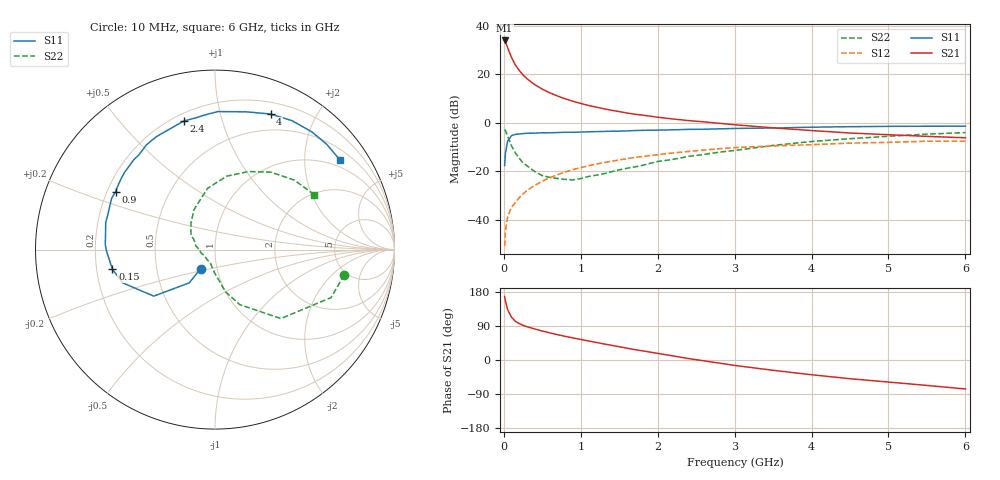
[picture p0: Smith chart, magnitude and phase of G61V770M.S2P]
! SIEMENS Small Signal Semiconductors
! BFG193
! Si NPN RF Bipolar Junction Transistor in SOT223
! VCE = 1.75 V  IC = 70 mA
! Common Emitter S-Parameters:  August  1996
# GHz  S  MA  R  50
!  f  S11  S21  S12  S22
! GHz  MAG  ANG  MAG  ANG  MAG  ANG  MAG  ANG
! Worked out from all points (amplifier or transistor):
!   36 points, 10 MHz to 6 GHz, reference 50 ohm
!   highest |S21| = 34.0 dB at 10 MHz (marker M1)
!   |S21| within 3 dB of that: start of sweep to 49.84 MHz
!   unconditionally stable (mu >= 1): start of sweep to 16.65 MHz; 183.1 MHz to 2.994 GHz; 3.017 GHz to 3.944 GHz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
!   at 250 MHz: K = 1.05, MAG = 23.1 dB, |S12| = -29.2 dB
!   at 1.4 GHz: K = 1.11, MAG = 8.5 dB, |S12| = -15.8 dB
!   at 6 GHz: K = 1.00, MAG = 0.6 dB, |S12| = -7.5 dB
!   S11 on the Smith chart (normalised r, x): 10 MHz: 0.83, -0.18; 150 MHz: 0.27, -0.09; 900 MHz: 0.23, +0.26; 2.4 GHz: 0.24, +0.76; 4 GHz: 0.32, +1.44; 6 GHz: 0.78, +2.93
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0.01  0.1328 -127.1  49.92 167.7  0.0029 71.7  0.7338 -11.1
0.02  0.2344 -127.7  46.95 156.9  0.0059 66.9  0.6994 -22.5
0.05  0.4286 -142.8  35.29 132.3  0.0118 64.6  0.5313 -46.3
0.1  0.5459 -160.1  22.21 112.9  0.0183 63.0  0.3363 -65.8
0.15  0.5823 -169.2  15.58 102.2  0.0231 64.3  0.2413 -76.2
0.2  0.5916 -174.6  12.03 96.2  0.0288 66.8  0.1881 -80.6
0.25  0.6049 -179.3  9.706 91.5  0.0345 67.4  0.1503 -86.4
0.3  0.612 177.4  8.155 87.9  0.0406 68.4  0.1314 -90.5
0.4  0.6164 171.6  6.173 82.0  0.0515 68.3  0.1001 -99.2
0.5  0.6271 166.2  4.956 76.3  0.0632 67.6  0.0822 -107.0
0.6  0.6279 162.0  4.15 71.4  0.0748 66.3  0.0754 -115.4
0.7  0.6341 157.8  3.576 66.7  0.0862 64.8  0.0717 -126.3
0.9  0.6414 149.8  2.791 58.2  0.1096 60.9  0.067 -148.0
1.1  0.6559 142.7  2.294 50.2  0.1312 56.9  0.079 -164.8
1.6  0.6856 126.1  1.601 31.2  0.184 45.4  0.1163 163.5
2.2  0.7213 108.9  1.204 10.7  0.2413 30.8  0.1777 139.1
2.4  0.7371 103.7  1.118 3.8  0.2582 26.5  0.2043 130.7
3.5  0.7871 77.2  0.792 -27.2  0.3362 -1.9  0.3443 96.8
4  0.8164 67.7  0.697 -38.9  0.357 -11.7  0.414 81.0
4.5  0.8368 59.1  0.62 -49.4  0.3841 -22.0  0.4736 66.7
5.5  0.8555 43.3  0.529 -67.1  0.4205 -45.1  0.5878 41.2
6  0.8567 35.6  0.494 -76.4  0.4203 -58.2  0.6319 28.9
